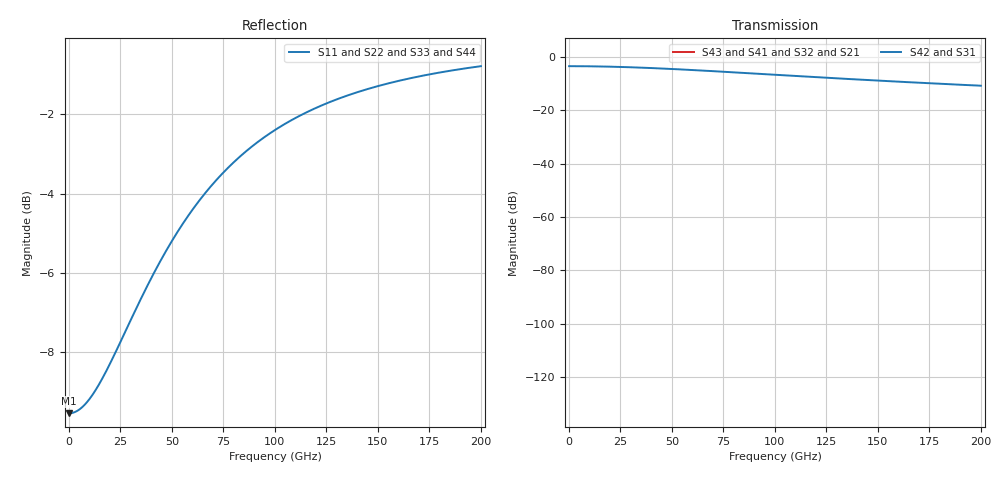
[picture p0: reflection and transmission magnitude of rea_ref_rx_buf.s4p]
! Created with skrf 1.10.0 (http://scikit-rf.org).
# Hz S RI R 50.0
!freq ReS11 ImS11 ReS12 ImS12 ReS13 ImS13
! ReS14 ImS14
! ReS21 ImS21 ReS22 ImS22 ReS23 ImS23
! ReS24 ImS24
! ReS31 ImS31 ReS32 ImS32 ReS33 ImS33
! ReS34 ImS34
! ReS41 ImS41 ReS42 ImS42 ReS43 ImS43
! ReS44 ImS44
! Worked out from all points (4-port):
!   2000 points, 100 MHz to 200 GHz, reference 50 ohm
!   strongest paths, dB at 100 MHz, 50.1 GHz, 100.1 GHz, 150.1 GHz, 200 GHz:
!     S42: -3.5, -4.6, -6.7, -8.9, -10.8
!     S31: -3.5, -4.6, -6.7, -8.9, -10.8
!     S43: -, -, -, -, -
!     S41: -, -, -, -, -
!     S32: -, -, -, -, -
!     S21: -, -, -, -, -
!   lowest |S11| = -9.5 dB at 100 MHz (marker M1), VSWR 2.00, Z = 25 - j0.0393 ohm
!   |S11| at or under -10 dB: nowhere
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1e8  -0.3333 -0.000698  0 0  0.6667 -0.000698  0 0
     0 0  -0.3333 -0.000698  0 0  0.6667 -0.000698
     0.6667 -0.000698  0 0  -0.3333 -0.000698  0 0
     0 0  0.6667 -0.000698  0 0  -0.3333 -0.000698
1.32e10  -0.3458 -0.0904  0 0  0.6542 -0.0904  0 0
         0 0  -0.3458 -0.0904  0 0  0.6542 -0.0904
         0.6542 -0.0904  0 0  -0.3458 -0.0904  0 0
         0 0  0.6542 -0.0904  0 0  -0.3458 -0.0904
3.72e10  -0.4212 -0.2255  0 0  0.5788 -0.2255  0 0
         0 0  -0.4212 -0.2255  0 0  0.5788 -0.2255
         0.5788 -0.2255  0 0  -0.4212 -0.2255  0 0
         0 0  0.5788 -0.2255  0 0  -0.4212 -0.2255
7.11e10  -0.5711 -0.3193  0 0  0.4289 -0.3193  0 0
         0 0  -0.5711 -0.3193  0 0  0.4289 -0.3193
         0.4289 -0.3193  0 0  -0.5711 -0.3193  0 0
         0 0  0.4289 -0.3193  0 0  -0.5711 -0.3193
9.98e10  -0.6814 -0.333  0 0  0.3186 -0.333  0 0
         0 0  -0.6814 -0.333  0 0  0.3186 -0.333
         0.3186 -0.333  0 0  -0.6814 -0.333  0 0
         0 0  0.3186 -0.333  0 0  -0.6814 -0.333
1.289e11  -0.7638 -0.3189  0 0  0.2362 -0.3189  0 0
          0 0  -0.7638 -0.3189  0 0  0.2362 -0.3189
          0.2362 -0.3189  0 0  -0.7638 -0.3189  0 0
          0 0  0.2362 -0.3189  0 0  -0.7638 -0.3189
2e11  -0.8762 -0.2592  0 0  0.1238 -0.2592  0 0
      0 0  -0.8762 -0.2592  0 0  0.1238 -0.2592
      0.1238 -0.2592  0 0  -0.8762 -0.2592  0 0
      0 0  0.1238 -0.2592  0 0  -0.8762 -0.2592
